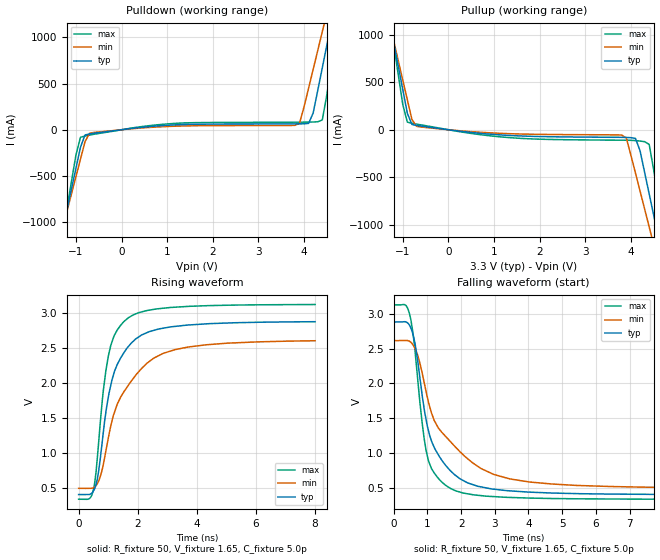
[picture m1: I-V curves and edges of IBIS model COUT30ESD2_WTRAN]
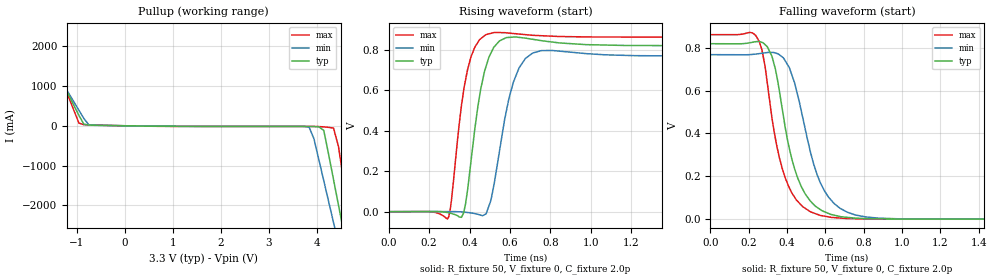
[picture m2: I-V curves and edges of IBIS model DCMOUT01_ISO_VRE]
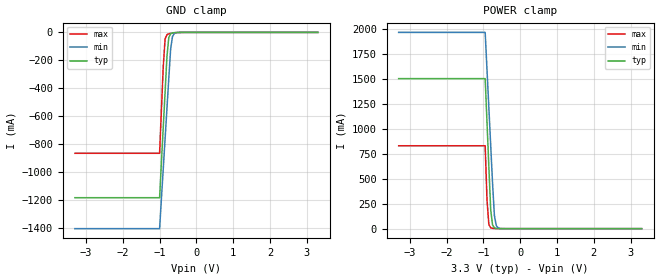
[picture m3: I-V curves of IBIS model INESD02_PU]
|   This file is an IBIS representation of the   |
|   Integrated Device Technology, Inc.   |
|   ICS841664I   |
|   FEMTOCLOCKS CRYSTAL-TO-HCSL CLOCK GENERATOR   |
[IBIS Ver]   4.1
[File name]   841664i_3v3.ibs
[File Rev]   1.0
[Date]   Oct  08   2008 | Last Modified
|   Oct  08   2008 | Generated
[Source] Originated at Integrated Device Technology, Inc.
[Disclaimer]
IDT hereby grants the user of this IBIS model a non-exclusive,
nontransferable license to use this IBIS model under the following terms.
Before using this IBIS model, the user should read this license.
If the user does not accept these terms,  the IBIS model should be
returned to IDT within 30 days.
   The user is granted this license only to use the IBIS model and
is not granted rights to sell, load, rent, lease or license the IBIS
model in whole or in part, or in modified form to anyone other than
user. User may modify the IBIS model to suit its specific
applications but rights to derivative works and such modifications
shall belong to IDT.
   This IBIS model is provided on an "AS IS" basis and IDT makes
absolutely no warranty with respect to the information contained
herein. IDT DISCLAIMS AND CUSTOMER WAIVES ALL WARRANTIES, EXPRESS
OR IMPLIED, INCLUDING WARRANTIES OF MERCHANTABILITY OR FITNESS FOR
A PARTICULAR PURPOSE. The entire risk as to quality and performance
is with the Customer. ACCORDINGLY, IN NO EVENT SHALL THE COMPANY BE
LIABLE FOR ANY DAMAGES, WHETHER IN CONTRACT OR TORT,INCLUDING ANY
LOST PROFITS OR OTHER INCIDENTAL, CONSEQUENTIAL, EXEMPLARY, OR
PUNITIVE DAMAGES ARISING OUT OF THE USE OR APPLICATION OF THE IBIS
model provided in this package. Further, IDT reserves the right to
make changes without notice to any product herein to improve
reliability, function, or design. IDT does not convey any license
under patent rights or any other intellectual property rights,
including those of third parties.
   IDT is not obligated to provide maintenance or support
for the licensed IBIS model.
[Copyright]   Copyright 2008 by Integrated Device Technology, Inc.
[Component]   841664GI
[Manufacturer] Integrated Devices Technology, INC.
[Package]
|TSSOP 28 Lead
|   typ   min   max
R_pkg   60.65m   52.4m   68.9m
L_pkg   1.989nH   1.431nH   2.547nH
C_pkg   0.314pF   0.254pF   0.374pF
[Pin]   signal_name   model_name   R_pin   L_pin   C_pin
1   VDD   POWER   68.9m   2.547n   0.374p
2   REF_OUT   COUT30ESD2_WTRAN   66.2m   2.360n   0.254p
3   GND   GND   63.4m   2.174n   0.334p
4   QA0   DCMOUT01_ISO_VRE   60.6m   1.988n   0.314p
5   nQA0   DCMOUT01_ISO_VRE   57.9m   1.802n   0.294p
6   VDDOA   POWER   55.1m   1.616n   0.274p
7   GND   GND   52.4m   1.431n   0.254p
8   QA1   DCMOUT01_ISO_VRE   52.4m   1.431n   0.254p
9   nQA1   DCMOUT01_ISO_VRE   55.1m   1.616n   0.274p
10   nREF_OE   INESD02_PU   57.9m   1.802n   0.294p
11   BYPASS   INESD02_PD   60.6m   1.988n   0.314p
12   REF_IN   INESD02_PD_PECL   63.4m   2.174n   0.334p
13   REF_SEL   INESD02_PD   66.2m   2.360n   0.254p
14   VDDA   POWER   68.9m   2.547n   0.374p
15   GND   GND   68.9m   2.547n   0.374p
16   XTAL_OUT   NC   66.2m   2.360n   0.254p
17   XTAL_IN   NC   63.4m   2.174n   0.334p
18   VDD   POWER   60.6m   1.988n   0.314p
19   MR_nOE   INESD02_PD   57.9m   1.802n   0.294p
20   nQB1   DCMOUT01_ISO_VRE   55.1m   1.616n   0.274p
21   QB1   DCMOUT01_ISO_VRE   52.4m   1.431n   0.254p
22   GND   GND   52.4m   1.431n   0.254p
23   VDDOB   POWER   55.1m   1.616n   0.274p
24   nQB0   DCMOUT01_ISO_VRE   57.9m   1.802n   0.294p
25   QB0   DCMOUT01_ISO_VRE   60.6m   1.988n   0.314p
26   FSEL1   INESD02_PD   63.4m   2.174n   0.334p
27   FSEL0   INESD02_PD   66.2m   2.360n   0.254p
28   IREF   NC   68.9m   2.547n   0.374p
[Diff Pin]  inv_pin  vdiff tdelay_typ tdelay_min  tdelay_max
4   5   NA   0   0   0
8   9   NA   0   0   0
21   20   NA   0   0   0
25   24   NA   0   0   0
| Models and submodels in the file (5): COUT30ESD2_WTRAN (Output), DCMOUT01_ISO_VRE (Open_source), INESD02_PU (Input), INESD02_PD (Input), INESD02_PD_PECL (Input)
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[Model]   COUT30ESD2_WTRAN
Model_type Output
Polarity  Non-Inverting
Vmeas= 1.65
Rref = 50
Cref = 0
Vref = 1.65
|Variable   typ   min   max
C_comp   2pF   1.5pF   2.5pF
[Voltage Range]   3.3   3.135   3.465
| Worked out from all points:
|   slope of the pulldown table from 0 to 0.495 V, typ, clamps not added: 17.2 ohm
|   slope of the pullup table from 0 to 0.495 V, typ, clamps not added: 17.5 ohm
|   rising waveform, R_fixture 50, V_fixture 1.65, C_fixture 5.0p: 20-80 % time 728ps typ, 1.2ns min, 484ps max; typ from 0.412 V to 2.88 V
|   falling waveform, R_fixture 50, V_fixture 1.65, C_fixture 5.0p: 20-80 % time 731ps typ, 1.36ns min, 421ps max; typ from 2.88 V to 0.411 V
[Pulldown]
|dc (V)   value(IS("/I77   value(IS("/I77   value(IS("/I77
-3.3V     -5.681A    -4.894A    -6.976A
-1.3V     -1.107A    -1.081A    -1.154A
-900mV    -189.9mA   -319.1mA   -81.68mA
-700mV    -45.08mA   -37.83mA   -57.92mA
3.9V      63.82mA    69.83mA    81.93mA
4.1V      68.79mA    451.5mA    82.63mA
4.2V      181.6mA    654.7mA    83.78mA
4.4V      671.1mA    1.062A     106.2mA
4.6V      1.163A     1.471A     695.2mA
4.7V      1.409A     1.676A     1.01A
4.8V      1.656A     1.881A     1.326A
6.6V      6.208A     5.657A     7.137A
[Pullup]
|  Voltage   I(typ)   I(min)   I(max)
-3.3V     6.157A     5.293A     7.58A
-1.3V     1.169A     1.142A     1.219A
-1V       421.7mA    521.2mA    264.2mA
-800mV    55.35mA    108.5mA    68.17mA
3.8V      -79.91mA   -56.07mA   -109.8mA
3.9V      -80.97mA   -89.22mA   -110.2mA
4.1V      -91.25mA   -456.4mA   -114.2mA
4.4V      -674.4mA   -1.021A    -154.3mA
4.6V      -1.129A    -1.399A    -716mA
4.7V      -1.356A    -1.588A    -1.006A
4.8V      -1.583A    -1.778A    -1.296A
6.6V      -5.678A    -5.19A     -6.516A
|  Voltage   I(typ)   I(min)   I(max)
[Ramp]
|   typ   min   max
dV/dt_r   1.493/1.2n   1.2/1.20n   1.666/1.20n
dV/dt_f   1.493/1.2n   1.2/1.20n   1.666/1.20n
[Rising Waveform]
R_fixture = 50
V_fixture = 1.65
V_fixture_max = 1.73
V_fixture_min = 1.57
C_fixture = 5.0p
| Time   typ   min   max
0s        412.2mV    501.6mV    346.3mV
499.3ps   460.7mV    509.8mV    475.1mV
671.9ps   726.5mV    600.5mV    1.12V
839.5ps   1.313V     847mV      1.905V
1.006ns   1.8V       1.221V     2.385V
1.3ns     2.258V     1.694V     2.752V
1.676ns   2.518V     1.966V     2.929V
2.303ns   2.718V     2.28V      3.033V
3.27ns    2.809V     2.478V     3.082V
8ns       2.875V     2.604V     3.12V
[Falling Waveform]
R_fixture = 50
V_fixture = 1.65
V_fixture_max = 1.73
V_fixture_min = 1.57
C_fixture = 5.0p
| Time   typ   min   max
0s        2.879V     2.613V     3.123V
361.2ps   2.882V     2.615V     3.117V
513.3ps   2.79V      2.588V     2.906V
836.7ps   1.866V     2.171V     1.471V
1.035ns   1.322V     1.727V     890mV
1.321ns   984.4mV    1.368V     646.7mV
1.846ns   682.6mV    1.085V     464.9mV
2.968ns   489.5mV    700.2mV    383.1mV
4.616ns   436mV      565.8mV    356.6mV
15ns      410.7mV    505.2mV    344.5mV
[Model]  DCMOUT01_ISO_VRE
Model_type Open_source
Polarity  Non-Inverting
Vmeas= .323
Rref = 50
Cref = 0
Vref = 0
|Variable   typ   min   max
C_comp   2p   1.5p   2.5p
|Variable   typ   min   max
[Voltage Range]   3.3   3.135   3.465
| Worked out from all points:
|   slope of the pullup table from 0 to 0.495 V, typ, clamps not added: 57.4 ohm
|   rising waveform, R_fixture 50, V_fixture 0, C_fixture 2.0p: 20-80 % time 68.9ps typ, 85.7ps min, 65.1ps max; typ from 0 V to 0.82 V
|   falling waveform, R_fixture 50, V_fixture 0, C_fixture 2.0p: 20-80 % time 119ps typ, 137ps min, 110ps max; typ from 0.82 V to 0 V
|  Voltage   I(typ)   I(min)   I(max)
[Pullup]
|  Voltage   I(typ)   I(min)   I(max)
-3.3V     5.929A     5.106A     7.3A
-2.075V   2.966A     2.639A     3.52A
-1.769V   2.226A     2.023A     2.576A
-952.6mV  259.6mA    387.7mA    67.22mA
-850.5mV  40.66mA    183.8mA    26.27mA
3.844V    -17.3mA    -33.95mA   -17.33mA
4.151V    -116.4mA   -1.378A    -29.1mA
4.355V    -1.355A    -2.431A    -58.99mA
4.559V    -2.622A    -3.486A    -1.33A
4.661V    -3.257A    -4.014A    -2.14A
4.763V    -3.891A    -4.542A    -2.95A
6.6V      -15.32A    -14.06A    -17.53A
[Ramp]
|   typ   min   max
dV/dt_r   0.824V/.4ns   .770V/.4ns   0.867V/.4ns
dV/dt_f   0.824V/.4ns   .770V/.4ns   0.867V/.4ns
R_load =   50.0000
[Rising Waveform]
R_fixture = 50
V_fixture = 0
C_fixture = 2.0p
| Time   typ   min   max
0s        1.402nV    4.01nV     367.5pV
297.2ps   -5.136mV   575uV      -25.12mV
370.9ps   -5.979mV   -1.874mV   596.9mV
426ps     405.7mV    -9.617mV   811.8mV
480.8ps   714mV      -11.24mV   874.1mV
506.1ps   783.3mV    56.91mV    880.7mV
547.7ps   842.7mV    298mV      884.4mV
616.9ps   862.1mV    638.7mV    879.5mV
713.2ps   851mV      783.6mV    870.8mV
2ns       819.7mV    768.5mV    861.9mV
[Falling Waveform]
R_fixture = 50
V_fixture = 0
C_fixture = 2.0p
| Time   typ   min   max
0s        819.6mV    768.4mV    861.9mV
236.8ps   829mV      771mV      858.6mV
297.2ps   805.7mV    778.4mV    636mV
339.5ps   701mV      776.1mV    376.7mV
389.8ps   433.6mV    741mV      195.1mV
455.5ps   192.6mV    579.7mV    82.79mV
521.7ps   84.34mV    315.8mV    33.94mV
616.9ps   25.88mV    102.3mV    10.07mV
756ps     4.142mV    19.3mV     1.608mV
2ns       287.7pV    5.065nV    462.5pV
[Model]   INESD02_PU
Model_type   Input
Polarity   Non-Inverting
Vinl = 0.80V
Vinh = 2.0V
|   typ   min   max
C_comp   2pF   1.5pF   2.5pF
|   typ   min   max
[Voltage range]  3.3V   3.15V   3.45V
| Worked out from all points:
|   GND clamp passes 1 mA (typ) near -0.56 V on its own axis
|   POWER clamp passes 1 mA (typ) near -0.61 V on its own axis
[GND_clamp]
|Voltage   I(typ)   I(min)   I(max)
-3.3V     -1.184A    -1.405A    -865.6mA
-1V       -1.184A    -1.405A    -865.6mA
-900mV    -678.5mA   -975.1mA   -244.1mA
-850mV    -426.2mA   -760.2mA   -46.92mA
-800mV    -174mA     -545.4mA   -16.17mA
-750mV    -37.03mA   -330.8mA   -9.981mA
-700mV    -9.767mA   -120.3mA   -7.122mA
-650mV    -3.616mA   -29.78mA   -4.922mA
-600mV    -1.7mA     -7.594mA   -3.115mA
-400mV    -123.9uA   -126uA     -173.9uA
3.3V      1.866nA    3.949uA    0A
[POWER_clamp]
|Voltage   I(typ)   I(min)   I(max)
-3.3V     1.506A     1.97A      832.1mA
-950mV    1.506A     1.97A      832.1mA
-900mV    1.063A     1.592A     287.2mA
-850mV    620.4mA    1.215A     41.77mA
-800mV    191.5mA    837.4mA    8.692mA
-750mV    37.69mA    460.1mA    3.262mA
-700mV    8.032mA    133.8mA    1.662mA
-650mV    2.005mA    32.58mA    840.1uA
-600mV    607uA      8.009mA    378.6uA
-450mV    33.11uA    139.8uA    23.88uA
3.3V      -71.13uA   -77.46uA   -62.11uA
